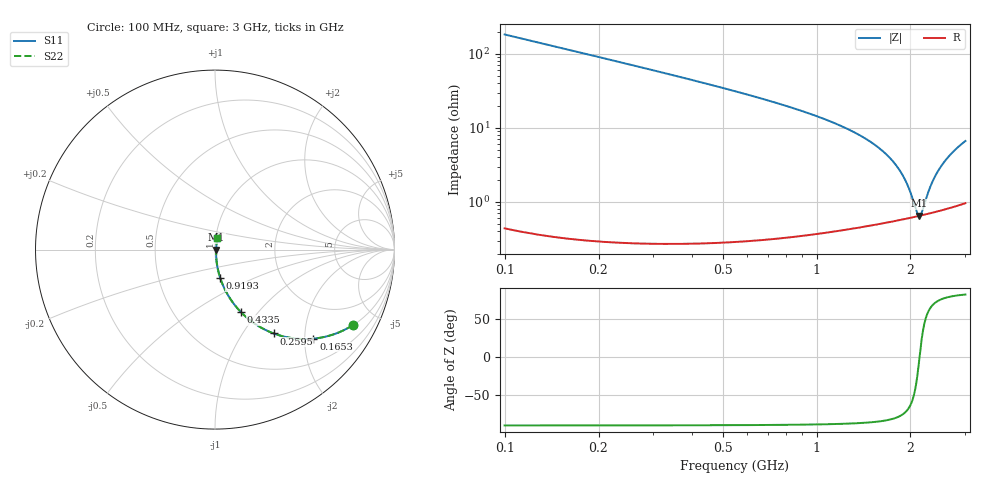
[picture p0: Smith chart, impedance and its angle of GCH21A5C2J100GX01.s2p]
!Murata Part Number: GCH21A5C2J100GX01
!These Parameters are Measured in Series Mode Connection
!Data Generated on Mar 13, 2026
!  o--ll--o
!Port1  Port2
!  o------o
!Operation Temp=25[degC], DC Bias Voltage=0[V]
!Freq. Start=100[MHz] Stop=3[GHz] 401[Steps]
# Hz S RI R 50
!Freq.(Hz) S11(Real) S11(Imag) S21(Real) S21(Imag) S12(Real) S12(Imag) S22(Real) S22(Imag)
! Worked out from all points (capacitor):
!   401 points, 100 MHz to 3 GHz, reference 50 ohm
!   read as one part in series: C = 8.69 pF near 114.5 MHz
!   lowest |Z| = 648 mohm at 2.137 GHz (marker M1)
!   series resonance near 2.139 GHz, so ESL is about 640 pH
!   S11 on the Smith chart (normalised r, x): 100 MHz: 1.01, -3.65; 165.2 MHz: 1.01, -2.20; 259.5 MHz: 1.01, -1.39; 433.5 MHz: 1.01, -0.81; 919.2 MHz: 1.01, -0.33; 3 GHz: 1.02, +0.13
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1e8  0.7689 -0.4203  0.2311 0.4203  0.2311 0.4203  0.7689 -0.4203
1.6525e8  0.548 -0.4963  0.452 0.4963  0.452 0.4963  0.548 -0.4963
2.0875e8  0.4304 -0.4935  0.5696 0.4935  0.5696 0.4935  0.4304 -0.4935
2.595e8  0.3266 -0.467  0.6734 0.467  0.6734 0.467  0.3266 -0.467
3.3925e8  0.2182 -0.4104  0.7818 0.4104  0.7818 0.4104  0.2182 -0.4104
4.335e8  0.1428 -0.3465  0.8572 0.3465  0.8572 0.3465  0.1428 -0.3465
5.8575e8  0.0797 -0.2659  0.9203 0.2659  0.9203 0.2659  0.0797 -0.2659
9.1925e8  0.0292 -0.158  0.9708 0.158  0.9708 0.158  0.0292 -0.158
1.0715e9  0.02 -0.1261  0.98 0.1261  0.98 0.1261  0.02 -0.1261
1.55e9  0.00813 -0.0566  0.9919 0.0566  0.9919 0.0566  0.00813 -0.0566
1.7095e9  0.00685 -0.0393  0.9931 0.0393  0.9931 0.0393  0.00685 -0.0393
1.84e9  0.00633 -0.0264  0.9937 0.0264  0.9937 0.0264  0.00633 -0.0264
1.94875e9  0.00619 -0.0164  0.9938 0.0164  0.9938 0.0164  0.00619 -0.0164
2.03575e9  0.00623 -0.00872  0.9938 0.00872  0.9938 0.00872  0.00623 -0.00872
2.101e9  0.00635 -0.00316  0.9937 0.00316  0.9937 0.00316  0.00635 -0.00316
2.13725e9  0.00644 -0.000132  0.9936 0.000132  0.9936 0.000132  0.00644 -0.000132
2.1735e9  0.00656 0.00286  0.9934 -0.00286  0.9934 -0.00286  0.00656 0.00286
2.275e9  0.00697 0.011  0.993 -0.011  0.993 -0.011  0.00697 0.011
2.3475e9  0.00736 0.0167  0.9926 -0.0167  0.9926 -0.0167  0.00736 0.0167
2.5215e9  0.00855 0.0299  0.9915 -0.0299  0.9915 -0.0299  0.00855 0.0299
2.73175e9  0.0105 0.0453  0.9895 -0.0453  0.9895 -0.0453  0.0105 0.0453
3e9  0.0137 0.0643  0.9863 -0.0643  0.9863 -0.0643  0.0137 0.0643
